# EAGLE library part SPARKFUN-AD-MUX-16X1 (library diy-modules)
SparkFun Analog/Digital MUX Breakout based on CD74HC4067 chip Source: https://www.sparkfun.com/products/9056
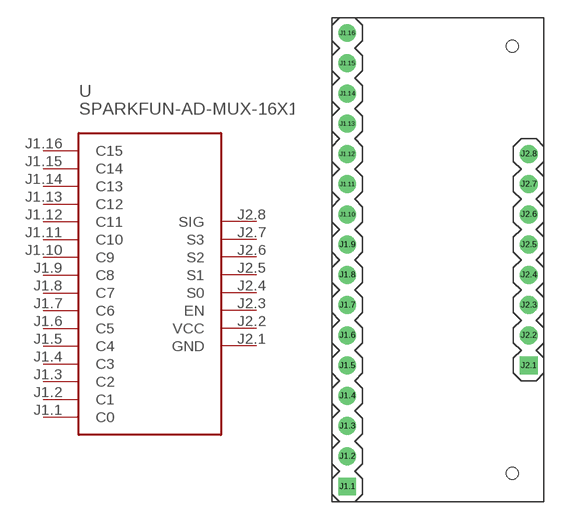
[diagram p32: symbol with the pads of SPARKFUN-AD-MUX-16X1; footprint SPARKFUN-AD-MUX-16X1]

Designator prefix -

## SPARKFUN-AD-MUX-16X1  [SPARKFUN-AD-MUX-16X1]
J1.1  C0
J1.2  C1
J1.3  C2
J1.4  C3
J1.5  C4
J1.6  C5
J1.7  C6
J1.8  C7
J1.9  C8
J1.10  C9
J1.11  C10
J1.12  C11
J1.13  C12
J1.14  C13
J1.15  C14
J1.16  C15
J2.1  GND  pwr
J2.2  VCC  pwr
J2.3  EN  in
J2.4  S0
J2.5  S1
J2.6  S2
J2.7  S3
J2.8  SIG

## Footprint SPARKFUN-AD-MUX-16X1 (pad centres in mm)
SparkFun Analog/Digital MUX Breakout based on CD74HC4067 chip
drill 1 square: J1.1 -7.62,-19.05; J2.1 7.62,-8.89
drill 1: J1.2 -7.62,-16.51; J1.3 -7.62,-13.97; J1.4 -7.62,-11.43; J1.5 -7.62,-8.89; J1.6 -7.62,-6.35; J1.7 -7.62,-3.81; J1.8 -7.62,-1.27; J1.9 -7.62,1.27; J1.10 -7.62,3.81; J1.11 -7.62,6.35; J1.12 -7.62,8.89; J1.13 -7.62,11.43; J1.14 -7.62,13.97; J1.15 -7.62,16.51; J1.16 -7.62,19.05; J2.2 7.62,-6.35; J2.3 7.62,-3.81; J2.4 7.62,-1.27; J2.5 7.62,1.27; J2.6 7.62,3.81; J2.7 7.62,6.35; J2.8 7.62,8.89
hole 1 at 6.245,-17.93
hole 1 at 6.245,17.93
